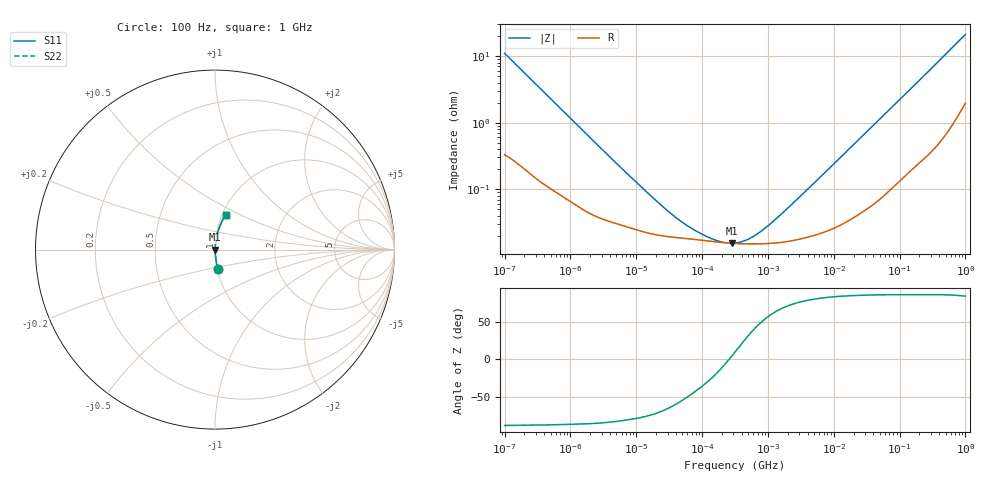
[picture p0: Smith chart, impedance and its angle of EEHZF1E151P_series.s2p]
!  *** S-Parameter ***
!  Copyright (C) Panasonic Industry
!  Conductive Polymer Hybrid Aluminum Electrolytic Capacitors
!  Parts No. EEHZF1E151P
!  Connection Mode : Series
!  1  o---||---o  2
!  GND o--------o GND
!  Conditions : Temperature = 20 degC , DC Bias = 0 V
! Frequency Range : 100Hz  -  1GHz  [ 401 Steps ]
# Hz S RI R 50
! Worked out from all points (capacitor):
!   401 points, 100 Hz to 1 GHz, reference 50 ohm
!   read as one part in series: C = 143 uF near 108.4 Hz
!   lowest |Z| = 15.4 mohm at 280.2 kHz (marker M1)
!   series resonance near 256.3 kHz, so ESL is about 2.7 nH
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100  0.0152 -0.1082  0.9848 0.1082  0.9848 0.1082  0.0152 -0.1082
108.3927  0.0133 -0.1002  0.9867 0.1002  0.9867 0.1002  0.0133 -0.1002
309.0295  0.00274 -0.0364  0.9973 0.0364  0.9973 0.0364  0.00274 -0.0364
1487.647  0.000569 -0.00789  0.9994 0.00789  0.9994 0.00789  0.000569 -0.00789
5854.637  0.000294 -0.00208  0.9997 0.00208  0.9997 0.00208  0.000294 -0.00208
22130.95  0.000203 -0.000581  0.9998 0.000581  0.9998 0.000581  0.000203 -0.000581
43903.59  0.000186 -0.000296  0.9998 0.000296  0.9998 0.000296  0.000186 -0.000296
83656.56  0.000174 -0.000152  0.9998 0.000152  0.9998 0.000152  0.000174 -0.000152
165958.7  0.000161 -5.41e-05  0.9998 5.41e-05  0.9998 5.41e-05  0.000161 -5.41e-05
220039.2  0.000156 -1.9e-05  0.9998 1.9e-05  0.9998 1.9e-05  0.000156 -1.9e-05
280220.6  0.000153 1.13e-05  0.9998 -1.13e-05  0.9998 -1.13e-05  0.000153 1.13e-05
316227.8  0.000153 2.69e-05  0.9998 -2.69e-05  0.9998 -2.69e-05  0.000153 2.69e-05
492606.3  0.000151 9.02e-05  0.9998 -9.02e-05  0.9998 -9.02e-05  0.000151 9.02e-05
831763.8  0.000151 0.00019  0.9998 -0.00019  0.9998 -0.00019  0.000151 0.00019
1522299  0.000158 0.000372  0.9998 -0.000372  0.9998 -0.000372  0.000158 0.000372
4704354  0.0002 0.00114  0.9998 -0.00114  0.9998 -0.00114  0.0002 0.00114
6.99842e7  0.00119 0.0157  0.9988 -0.0157  0.9988 -0.0157  0.00119 0.0157
1.631173e8  0.00332 0.0354  0.9967 -0.0354  0.9967 -0.0354  0.00332 0.0354
3.235937e8  0.0086 0.0684  0.9914 -0.0684  0.9914 -0.0684  0.0086 0.0684
5.688529e8  0.0219 0.1173  0.9781 -0.1173  0.9781 -0.1173  0.0219 0.1173
9.225714e8  0.0516 0.1818  0.9484 -0.1818  0.9484 -0.1818  0.0516 0.1818
1e9  0.0595 0.1946  0.9405 -0.1946  0.9405 -0.1946  0.0595 0.1946
